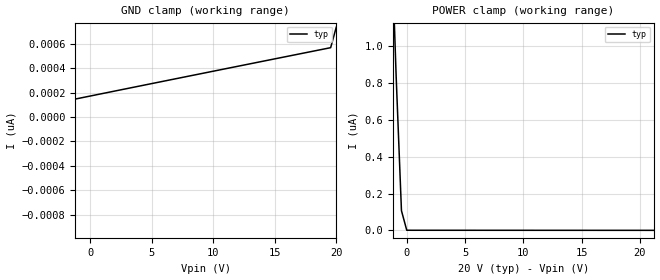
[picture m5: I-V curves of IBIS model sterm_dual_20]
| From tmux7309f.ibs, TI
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| sterm_dual_20
[Model]   sterm_dual_20
Model_type   Terminator
|   typ   min   max
C_comp   1.598234e-12   NA   NA
[Voltage Range]   20   NA   NA
[Temperature Range]   27   NA   NA
[Power Clamp Reference]   20   NA   NA
[GND Clamp Reference]   0   NA   NA
[GND Clamp]
|   Voltage   I(typ)   I(min)   I(max)
-25V      -20.05uA   NA         NA
-20.45V   -10.62uA   NA         NA
-20V      -640.5pA   NA         NA
-19.55V   -233.3pA   NA         NA
19.55V    568.6pA    NA         NA
20V       736pA      NA         NA
[POWER Clamp]
|   Voltage   I(typ)   I(min)   I(max)
-5V       8.864uA    NA         NA
-1.364V   1.681uA    NA         NA
-909.1mV  835.3nA    NA         NA
-454.5mV  106.8nA    NA         NA
0V        736pA      NA         NA
40V       -640.5pA   NA         NA
